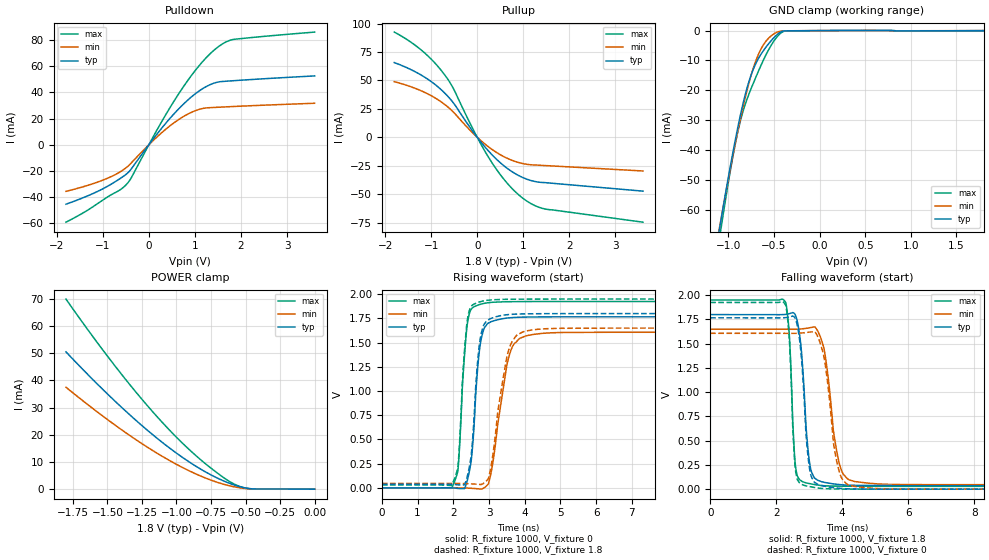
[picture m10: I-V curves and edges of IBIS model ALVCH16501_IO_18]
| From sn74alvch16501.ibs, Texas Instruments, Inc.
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[Model]   ALVCH16501_IO_18
Model_type  I/O
Vinl=0.5775
Vinh=1.2675
Enable   Active-Low
Vref =   0
Rref =   1000
Cref =   30p
Vmeas =   0.9
| variable   typ   min   max
C_comp   3.16pF   2.60pF   3.42pF
| C_pullup   4.37pF   3.25pF   5.20pF
| C_pulldown   3.83pF   2.58pF   5.29pF
| C_tri-state   3.16pF   2.60pF   3.42pF
[Temperature Range]   40   100   -40
| Ambient temperature   25   85   -40
[Voltage range]   1.8   1.65   1.95
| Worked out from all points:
|   slope of the pulldown table from 0 to 0.27 V, typ, clamps not added: 21.9 ohm
|   slope of the pullup table from 0 to 0.27 V, typ, clamps not added: 20.5 ohm
|   GND clamp passes 1 mA (typ) near -0.45 V on its own axis
|   POWER clamp passes 1 mA (typ) near -0.55 V on its own axis
|   rising waveform, R_fixture 1000, V_fixture 0: 20-80 % time 208ps typ, 377ps min, 182ps max; typ from 0 V to 1.77 V
|   falling waveform, R_fixture 1000, V_fixture 1.8: 20-80 % time 213ps typ, 343ps min, 143ps max; typ from 1.8 V to 0.037 V
|   rising waveform, R_fixture 1000, V_fixture 1.8: 20-80 % time 205ps typ, 371ps min, 179ps max; typ from 0.037 V to 1.8 V
|   falling waveform, R_fixture 1000, V_fixture 0: 20-80 % time 210ps typ, 329ps min, 142ps max; typ from 1.77 V to 0 V
[GND Clamp]
| ALVCH16501_IO_18
|   Voltage   I(typ)   I(min)   I(max)
-1.8V     -206mA     -196.5mA   -223.2mA
-1.09V    -64.93mA   -64.63mA   -67.98mA
-1.075V   -62.21mA   -62.07mA   -65.01mA
-970mV    -43.95mA   -44.8mA    -45.39mA
-905mV    -33.61mA   -34.82mA   -35.05mA
-850mV    -25.77mA   -26.97mA   -28.11mA
-785mV    -18.07mA   -18.71mA   -22.06mA
-715mV    -12.06mA   -11.45mA   -16.75mA
-645mV    -8.018mA   -6.288mA   -11.79mA
-490mV    -2.005mA   -884.9uA   -2.998mA
-375mV    -79.77uA   -87.66uA   -123.4uA
1.8V      922.9pA    18.22uA    -33.66uA
[POWER Clamp]
| ALVCH16501_IO_18
|   Voltage   I(typ)   I(min)   I(max)
-1.8V     50.51mA    37.5mA     69.93mA
-1.49V    34.56mA    25.25mA    48.3mA
-1.345V   27.67mA    19.99mA    38.91mA
-1.21V    21.65mA    15.43mA    30.68mA
-1.08V    16.3mA     11.4mA     23.32mA
-960mV    11.81mA    8.063mA    17.09mA
-845mV    7.986mA    5.272mA    11.7mA
-725mV    4.596mA    2.87mA     6.736mA
-600mV    1.86mA     1.051mA    2.341mA
-495mV    387.5uA    210.7uA    356.3uA
-435mV    84.99uA    88.28uA    117.3uA
-16.28fV  922.9pA    48.41nA    27.85pA
[Pulldown]
| ALVCH16501_IO_18
|   Voltage   I(typ)   I(min)   I(max)
-1.8V     -45.43mA   -35.61mA   -59.18mA
-970mV    -33.11mA   -26.63mA   -41.58mA
-620mV    -25.73mA   -20.63mA   -34.33mA
-470mV    -21.87mA   -16.88mA   -29.66mA
-380mV    -18.4mA    -13.77mA   -25.14mA
190mV     8.78mA     6.409mA    12.19mA
660mV     27.89mA    19.59mA    39.62mA
1.105V    41.45mA    27.19mA    61.03mA
1.49V     47.86mA    28.67mA    74.47mA
1.675V    48.58mA    28.99mA    78.59mA
1.85V     49.01mA    29.28mA    80.62mA
3.6V      52.64mA    31.74mA    86.15mA
[Pullup]
| ALVCH16501_IO_18
|   Voltage   I(typ)   I(min)   I(max)
-1.8V     65.65mA    48.88mA    92.48mA
-1.215V   54.66mA    40.83mA    76.71mA
-970mV    48.1mA     35.89mA    67.5mA
-745mV    40.44mA    30.03mA    56.93mA
-530mV    30.9mA     22.63mA    43.79mA
-40mV     2.168mA    1.54mA     3.114mA
290mV     -14.05mA   -9.788mA   -20.45mA
640mV     -26.96mA   -18.28mA   -39.88mA
990mV     -35.44mA   -23.14mA   -53.58mA
1.235V    -38.74mA   -24.38mA   -59.76mA
1.48V     -39.94mA   -24.91mA   -63.15mA
3.6V      -47.41mA   -29.67mA   -74.71mA
[Ramp]
| ALVCH16501_IO_18
| variable   typ   min   max
dV/dt_r   1.06/2.18E-10   0.97/4.15E-10   1.16/1.96E-10
dV/dt_f   1.07/2.21E-10   0.98/3.72E-10   1.16/1.46E-10
R_load = 1000
[Rising Waveform]
| ALVCH16501_IO_18
R_fixture =   1000
C_fixture =   0
L_fixture =   0
V_fixture =   0
V_fixture_min = 0
V_fixture_max = 0
|   Time   V(typ)   V(min)   V(max)
0s        73.93pV    3.457nV    56.1pV
1.95ns    728.4uV    1.388mV    -1.578mV
2.13ns    -6.26mV    1.012mV    174.9mV
2.315ns   -7.258mV   -731.6uV   1.371V
2.5ns     273.8mV    -4.37mV    1.841V
2.755ns   1.482V     -12.66mV   1.895V
3.01ns    1.706V     76.83mV    1.914V
3.61ns    1.757V     1.417V     1.923V
4.495ns   1.766V     1.596V     1.925V
50ns      1.767V     1.607V     1.925V
[Falling Waveform]
| ALVCH16501_IO_18
R_fixture =   1000
C_fixture =   0
L_fixture =   0
V_fixture =   1.8
V_fixture_min = 1.65
V_fixture_max = 1.95
|   Time   V(typ)   V(min)   V(max)
0s        1.8V       1.65V      1.95V
2.29ns    1.802V     1.649V     1.924V
2.4ns     1.81V      1.649V     1.582V
2.56ns    1.809V     1.649V     332.2mV
2.75ns    1.478V     1.652V     88.15mV
3.01ns    276mV      1.664V     57.59mV
3.32ns    83.68mV    1.586V     39.55mV
3.955ns   46.09mV    215.7mV    30.77mV
4.81ns    38mV       60.96mV    29.43mV
50ns      37.13mV    45.98mV    29.27mV
[Rising Waveform]
| ALVCH16501_IO_18
R_fixture =   1000
C_fixture =   0
L_fixture =   0
V_fixture =   1.8
V_fixture_min = 1.65
V_fixture_max = 1.95
|   Time   V(typ)   V(min)   V(max)
0s        37.13mV    45.98mV    29.27mV
1.95ns    37.41mV    46.87mV    28.13mV
2.13ns    30.84mV    46.23mV    209.4mV
2.315ns   31.71mV    44.43mV    1.424V
2.5ns     327.6mV    41.2mV     1.872V
2.745ns   1.518V     35.15mV    1.921V
3ns       1.74V      120.2mV    1.939V
3.565ns   1.79V      1.439V     1.948V
4.37ns    1.799V     1.638V     1.95V
50ns      1.8V       1.65V      1.95V
[Falling Waveform]
| ALVCH16501_IO_18
R_fixture =   1000
C_fixture =   0
L_fixture =   0
V_fixture =   0
V_fixture_min = 0
V_fixture_max = 0
|   Time   V(typ)   V(min)   V(max)
0s        1.767V     1.607V     1.925V
2.29ns    1.769V     1.607V     1.895V
2.4ns     1.776V     1.607V     1.537V
2.555ns   1.774V     1.606V     307.3mV
2.75ns    1.413V     1.61V      55.93mV
3ns       235.7mV    1.619V     27.69mV
3.3ns     45.2mV     1.54V      10.16mV
3.925ns   8.642mV    165.9mV    1.504mV
4.745ns   844.6uV    13.88mV    164.6uV
50ns      2.576nV    10.01nV    368.4pV
